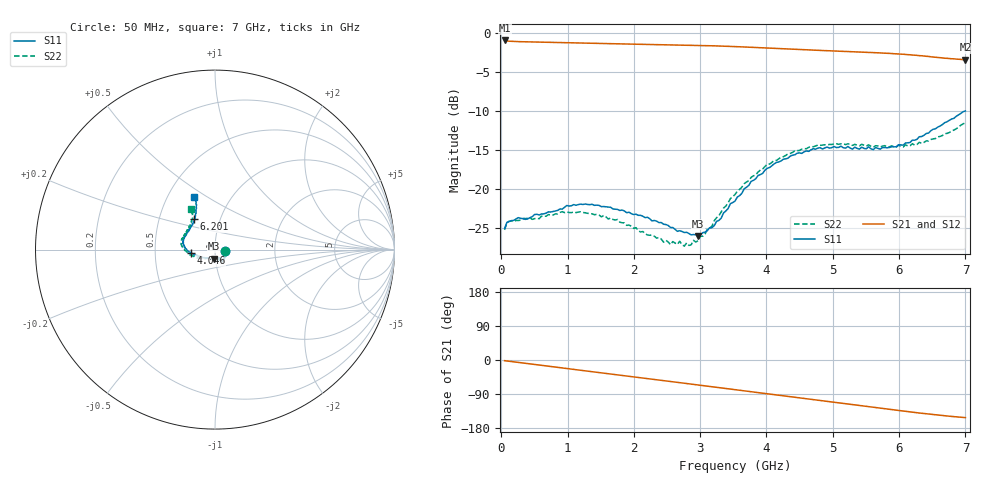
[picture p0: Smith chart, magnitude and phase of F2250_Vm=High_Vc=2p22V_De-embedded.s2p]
! Integrated Device Technology
! Corporate Headquarters
! 6024 Silver Creek Valley Road
! San Jose, CA 95138  USA
! Phone:  1-408-284-8200
! Toll Free:  1-800-223-1366
! Webpage:  http://www.idt.com/
! Timing and RF Division
! 515 Groton Road, Suite 102
! Westford, MA 01886-6024
! Device:  F2250
! Description: Voltage Variable RF Attenuator
! Frequency:  50.0 -  6000.00 MHz
! Package:  3x3 mm Thin QFN Plastic Package: 16 pin
! Ports:  2 RF, 3 DC
!  Pin  1  = GND
!  Pin  2  = NC
!  Pin  3  = RF1  = Port 1
!  Pin  4  = NC
!  Pin  5  = GND
!  Pin  6  = GND
!  Pin  7  = GND
!  Pin  8  = GND
!  Pin  9  = NC
!  Pin 10  = RF2  = Port 2
!  Pin 11  = NC
!  Pin 12  = GND
!  Pin 13  = GND
!  Pin 14  = VCNTRL
!  Pin 15  = VDD
!  Pin 16  = VMODE
! Vcntrl:  2.220 Volts
! Vmode:  +3.300 Volts
! Vdd:  +3.30  Volts
! Current:  1.316 mA
! Data:  The device was measured on a the F2250 evaluation board which has
!  individual transmission lines to the RF pins.  Data was collected
!  using a calibrated network analyzer.  The evaluation board was
!  de-embedded using a TRL calibration technique.
!  The reference plane is the edge of the package pin.
! Misc:  SN 10
!  Action Tracker AT0258
! Date Measured:  2014-11-26
! Date:  2015-10-15  MJV
! Note:
!  Integrated Device Technology supplies this data as a sample of measured
!  data at the package pin for this product.  Your particular data for this
!  product may vary.
!  Data was taken at 25 degrees C.
!  Integrated Device Technology reserves the right to change this data at anytime.
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# GHz S dB R 50
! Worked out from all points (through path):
!   201 points, 50 MHz to 7 GHz, reference 50 ohm
!   highest |S21| = -0.92 dB at 50 MHz (marker M1); lowest = -3.4 dB at 7 GHz (marker M2)
!   group delay of S21, straight-line fit = 61.1 ps
!   lowest |S11| = -26.1 dB at 2.969 GHz (marker M3), VSWR 1.10, Z = 49.4 - j4.92 ohm
!   |S11| at or under -10 dB: start of sweep to 6.996 GHz
!   |S22| runs from -27.4 to -11.5 dB; largest |S21 - S12| = 0.0019
!   S11 on the Smith chart (normalised r, x): 50 MHz: 1.12, -0.02; 4.046 GHz: 0.76, -0.03; 6.201 GHz: 0.75, +0.27; 7 GHz: 0.68, +0.44
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0.05  -25.11 -10.0  -0.92 -1.8  -0.92 -1.8  -25.28 -10.4
0.1195  -24.21 -9.7  -1.02 -3.2  -1.02 -3.2  -24.18 -8.6
0.91875  -22.62 -48.4  -1.21 -21.0  -1.21 -21.1  -22.94 -50.0
1.2315  -22.02 -56.2  -1.27 -27.9  -1.27 -27.9  -23.06 -60.5
1.75275  -22.65 -63.0  -1.37 -39.1  -1.37 -39.1  -23.95 -67.2
2.37825  -24.35 -63.0  -1.46 -52.8  -1.46 -52.8  -26.26 -67.6
2.552  -24.97 -67.7  -1.48 -56.6  -1.48 -56.7  -27.18 -74.2
2.691  -25.40 -75.3  -1.51 -59.7  -1.51 -59.8  -26.75 -81.6
2.7605  -25.63 -77.4  -1.52 -61.3  -1.52 -61.3  -27.38 -86.1
2.969  -26.05 -94.6  -1.56 -66.0  -1.56 -66.0  -26.68 -104.7
3.21225  -24.74 -124.4  -1.62 -71.5  -1.62 -71.5  -24.10 -129.4
3.4555  -21.91 -145.9  -1.69 -76.9  -1.69 -77.0  -21.26 -144.7
3.525  -21.59 -150.3  -1.71 -78.5  -1.71 -78.5  -20.74 -148.0
3.76825  -19.05 -163.0  -1.81 -84.0  -1.81 -84.0  -18.53 -159.0
4.04625  -17.27 -172.6  -1.92 -90.2  -1.92 -90.2  -16.82 -169.5
4.4285  -15.63 177.1  -2.06 -98.6  -2.07 -98.6  -15.11 179.1
4.7065  -14.85 170.1  -2.16 -104.8  -2.17 -104.8  -14.60 173.3
5.054  -14.70 161.9  -2.29 -112.5  -2.29 -112.5  -14.20 166.2
5.85325  -14.69 135.9  -2.59 -130.0  -2.59 -130.1  -14.61 147.4
6.20075  -13.74 124.3  -2.80 -137.7  -2.80 -137.8  -14.20 138.4
6.54825  -12.29 116.1  -3.07 -144.7  -3.07 -144.8  -13.54 127.0
7  -9.99 111.2  -3.40 -152.1  -3.41 -152.2  -11.52 120.7
